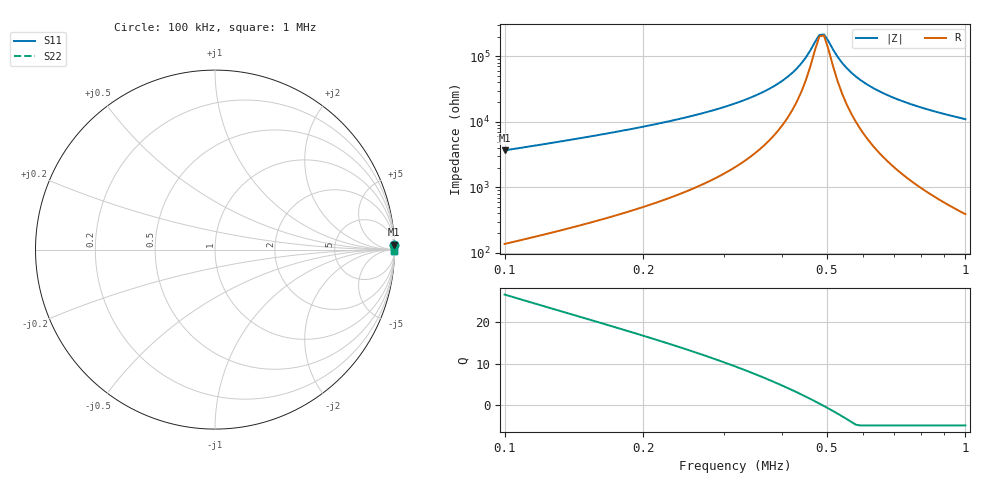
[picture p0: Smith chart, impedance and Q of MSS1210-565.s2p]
# MHz S MA R 50
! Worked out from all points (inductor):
!   102 points, 100 kHz to 1 MHz, reference 50 ohm
!   read as one part in series: L = 5.58 mH near 100 kHz
!   highest Q = 26.8 at 100 kHz (marker M1), where L = 5.84 mH
!   self-resonance near 482.1 kHz
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0.1  0.9986 1.6  0.02721 -86.3  0.02721 -86.3  0.9986 1.6
0.1256059  0.9989 1.2  0.02112 -86.4  0.02112 -86.4  0.9989 1.2
0.1577683  0.9991 0.9  0.01613 -86.2  0.01613 -86.2  0.9991 0.9
0.2546482  0.9993 0.5  0.008139 -85.2  0.008139 -85.2  0.9993 0.5
0.3424944  0.9995 0.2  0.004241 -82.5  0.004241 -82.5  0.9995 0.2
0.3751953  0.9995 0.2  0.003136 -80.4  0.003136 -80.4  0.9995 0.2
0.4017542  0.9995 0.1  0.00233 -77.6  0.00233 -77.6  0.9995 0.1
0.4204965  0.9995 0.1  0.001804 -74.4  0.001804 -74.4  0.9995 0.1
0.4401132  0.9995 0.1  0.001293 -68.5  0.001293 -68.5  0.9995 0.1
0.4502621  0.9995 0.1  0.001047 -63.4  0.001047 -63.4  0.9995 0.1
0.4821346  0.9995 0.0  0.0004725 -17.1  0.0004725 -17.1  0.9995 0.0
0.4932525  0.9996 -0.0  0.0004641 15.8  0.0004641 15.8  0.9996 -0.0
0.5281682  0.9996 -0.1  0.00102 64.9  0.00102 64.9  0.9996 -0.1
0.5403477  0.9996 -0.1  0.001265 70.2  0.001265 70.2  0.9996 -0.1
0.5528079  0.9996 -0.1  0.001517 73.8  0.001517 73.8  0.9996 -0.1
0.5785971  0.9996 -0.1  0.002037 78.2  0.002037 78.2  0.9996 -0.1
0.6195541  0.9996 -0.2  0.002836 81.7  0.002836 81.7  0.9996 -0.2
0.6634103  0.9996 -0.2  0.003655 83.7  0.003655 83.7  0.9996 -0.2
0.7103709  0.9996 -0.3  0.004493 85.0  0.004493 85.0  0.9996 -0.3
0.7781962  0.9996 -0.3  0.005647 86.0  0.005647 86.0  0.9996 -0.3
0.8524974  0.9996 -0.4  0.006849 86.7  0.006849 86.7  0.9996 -0.4
1  0.9996 -0.5  0.009098 87.4  0.009098 87.4  0.9996 -0.5
